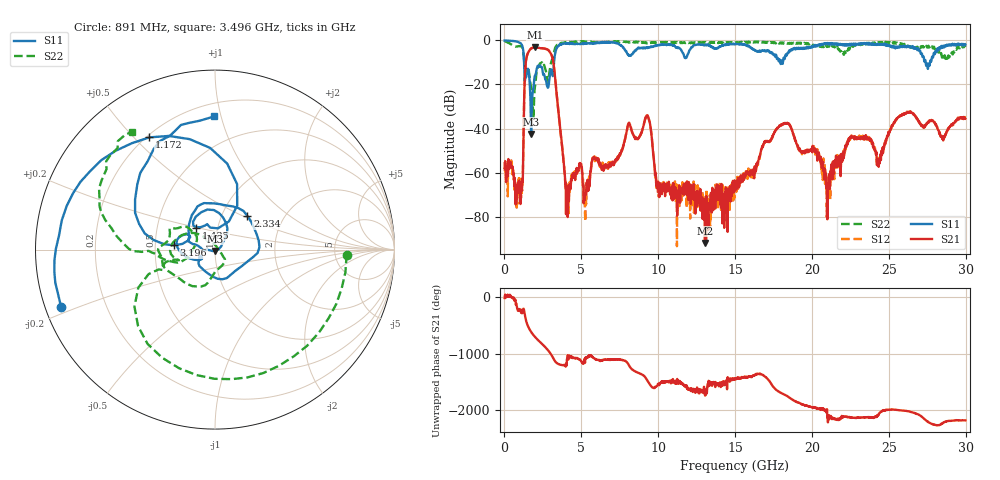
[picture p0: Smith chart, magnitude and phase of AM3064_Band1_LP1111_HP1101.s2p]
# Hz S DB R 50.0
!freq dBS11 angS11 dBS21 angS21 dBS12 angS12 dBS22 angS22
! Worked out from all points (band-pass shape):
!   1600 points, 10 MHz to 29.98 GHz, reference 50 ohm
!   highest |S21| = -3.21 dB at 2.016 GHz (marker M1); lowest = -91.9 dB at 13.04 GHz (marker M2)
!   |S21| within 3 dB of the highest: 1.5 GHz to 3.032 GHz (1.532 GHz wide, 67.6 % of centre)
!   lowest |S11| = -42.5 dB at 1.734 GHz (marker M3), VSWR 1.02, Z = 50 - j0.752 ohm
!   |S11| at or under -10 dB: 1.277 GHz to 3.225 GHz (1.949 GHz wide, 86.6 % of centre); 17.94544 GHz to 17.99523 GHz (49.79 MHz wide, 0.277 % of centre); 27.4 GHz to 27.68 GHz (282.2 MHz wide, 1.02 % of centre)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
!   |S22| runs from -35.5 to -0.2 dB; largest |S21 - S12| = 0.012
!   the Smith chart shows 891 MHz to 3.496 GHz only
!   S11 on the Smith chart (normalised r, x): 891 MHz: 0.05, -0.18; 1.172 GHz: 0.21, +0.55; 1.435 GHz: 0.79, +0.20; 2.334 GHz: 1.32, +0.53; 3.196 GHz: 0.63, +0.03; 3.496 GHz: 0.29, +0.95
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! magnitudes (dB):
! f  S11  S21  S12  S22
! 10 MHz  -0.1  -57.9  -55.2  -0.2
! 891 MHz  -0.8  -69.1  -69.5  -2.7
! 1.172 GHz  -2.8  -62.7  -63.2  -3.5
! 1.435 GHz  -15.8  -7.8  -7.8  -13.6
! 1.734 GHz  -42.5  -3.8  -3.7  -21.3
! 2.016 GHz  -15.8  -3.2  -3.2  -19.3
! 2.334 GHz  -11.7  -3.6  -3.5  -10.4
! 3.196 GHz  -12.7  -10.7  -10.5  -6.4
! 3.496 GHz  -2.6  -31.6  -31.6  -1.9
! 4.059 GHz  -1.4  -75.0  -75.2  -0.8
! 5.015 GHz  -1.4  -57.2  -56.5  -0.5
! 9.288 GHz  -3.5  -34.1  -34.1  -1.3
! 10 GHz  -2.2  -64.0  -65.9  -0.9
! 13.04 GHz  -2.2  -91.9  -73.4  -1.0
! 15 GHz  -1.6  -67.4  -66.2  -1.1
! 18 GHz  -9.6  -38.1  -38.3  -1.5
! 19.99 GHz  -3.3  -49.4  -50.0  -1.7
! 21.06 GHz  -1.8  -66.2  -62.5  -2.1
! 22.47 GHz  -1.5  -43.9  -43.6  -3.7
! 24.34 GHz  -2.0  -57.3  -54.6  -1.1
! 25 GHz  -2.0  -42.7  -42.3  -1.1
! 29.98 GHz  -1.8  -35.5  -34.9  -2.9
